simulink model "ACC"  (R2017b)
settings: Solver=FixedStepDiscrete  StartTime=0.0  StopTime=10.0  FixedStep=0.01  RelTol=1e-3  EnableMultiTasking=on
undefined symbols (not defined in the file): ACC_CONST0_NUMB, ACC_CONST1000_NUMB, ACC_CONST100_NUMB, ACC_CONST121_NUMB, ACC_CONST1_NUMB, ACC_CONST2047_NUMB, ACC_CONST60000_NUMB, ACC_CONST60_NUMB, ACC_CONSTF1_NUMB, ACC_RUNTIME_MS, ASWTYPE_FALSE, ASWTYPE_TRUE, CcACC_ACChrgDispSOCPrmt_pct, CcACC_ACChrgMismatch_ms, CcACC_ACChrgPACKVolLim_V, CcACC_ACChrgPACKVolLimTi_ms, CcACC_ACChrgPrmtObcFltLvl_numb, CcACC_ACChrgPrmtVcuFltLvl_numb, CcACC_ACChrgStepCurr_A, CcACC_ACChrgTempPrmtDelayTime_ms, CcACC_ACCrntUnctrolTi_ms, CcACC_ACFullChrgHysVolt_mV, CcACC_ACFullStepChrgTi1_ms, CcACC_ACFullStepChrgTi2_ms, CcACC_ACMaxChrgCurr_A, CcACC_ACStepChrgWaitTime_ms, CcACC_ACStop2DefaultTi_ms, CcACC_ACStop2DefaultTiDelay_ms, CcACC_BatFullResetTime_ms, CcACC_ChrgCrnt0HysVolt_mV, CcACC_ChrgEndDeviationVol1_mV, CcACC_ChrgEndDeviationVol2_mV, CcACC_ChrgEndDeviationVol3_mV, CcACC_ChrgMaxPackVoltLimt_V, CcACC_ChrgPwr1_W, CcACC_ChrgPwr2_W, CcACC_ChrgPwr3_W, CcACC_ChrgSt2StepChrgDeviVol_mV, CcACC_ChrgSt2StepChrgTime_ms, CcACC_ChrgStCutoffTime_ms, CcACC_ChrgStFullChrgCrnt_A, CcACC_CPDutyLowThrhd_pct, CcACC_CrntFilterTi1_cnt, CcACC_CrntFilterTi2_cnt, CcACC_CrntFilterTi2_ms, CcACC_CurrObcPreHeatLowThrhd_A, CcACC_DiffACChrgCrnt_A, CcACC_DiffACChrgCrntTi_ms, CcACC_DispSOCCalStart_pct, CcACC_DispSOCDiff_pct, CcACC_ElecLckRemTimeHold_ms, CcACC_HeatChrgCrnt0Time_ms, CcACC_HeatChrgCrnt1Time_ms, CcACC_Initial500Ti_ms, CcACC_Initial700Ti_ms, CcACC_MaxACChrgCellTemp_C, CcACC_MaxPackVoltLimt_V, CcACC_MinACChrgCellTemp_C, CcACC_MinACChrgCrntRqst_A, CcACC_OBCChrgPwr_W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
libraries: AIWAYS_Powertrain_BMS_lib x94, simulink x2
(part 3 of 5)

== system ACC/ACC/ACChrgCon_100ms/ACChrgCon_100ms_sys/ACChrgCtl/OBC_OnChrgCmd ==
  LbACC_ObcChrgCmd_flg : Inport
  GbADP_ChrgStopActive_flg : Inport  Port=2
  GeACC_ACChrgState_enum : Inport  Port=3
  GeUDS_AreaSel_enum : Inport  Port=4
  ACC_GbACC_ObcChrgCmd_flg : AIWAYS_Powertrain_BMS_lib/Signals/OverWrite  OverWrite_Value=CbACC_ObcChrgCmdOvr_flg  OverWrite_flag=CbACC_ObcChrgCmdOvrSwt_flg
  BMSDelay : AIWAYS_Powertrain_BMS_lib/Debounce & Delay/BMSDelay
  Constant1 : Constant  Value=ASWTYPE_FALSE
  Constant2 : Constant  Value=CcACC_ObcOnChrgCmdTi_ms
  Constant3 : Constant  Value=ASWTYPE_FALSE
  Constant4 : Constant  Value=Enum_ACCACChrgState.Enum_ACCACChrgState_Default
  Constant5 : Constant  Value=ACC_RUNTIME_MS
  Constant6 : Constant  Value=Enum_ACCACChrgState.Enum_ACCACChrgState_Stop
  Constant7 : Constant  Value=Enum_UDSAreaSel.Enum_UDSAreaSel_EU
  Constant8 : Constant  Value=ASWTYPE_FALSE
  Data Type Conversion1 : DataTypeConversion
  EdgeRising : AIWAYS_Powertrain_BMS_lib/Logical Operators/EdgeRising
  Logical Operator : Logic  Operator=OR  AllPortsSameDT=off  OutDataTypeStr=boolean
  Logical Operator1 : Logic  Operator=OR  Inputs=3  AllPortsSameDT=off  OutDataTypeStr=boolean
  Relational Operator1 : RelationalOperator  Operator===  OutDataTypeStr=boolean
  Relational Operator2 : RelationalOperator  Operator===  OutDataTypeStr=boolean
  Relational Operator3 : RelationalOperator  Operator===  OutDataTypeStr=boolean
  Switch : Switch  Criteria=u2 ~= 0  Threshold=1  RndMeth=Zero
  Switch1 : Switch  Criteria=u2 ~= 0  Threshold=1  RndMeth=Zero
  Switch3 : Switch  Criteria=u2 ~= 0  Threshold=1  RndMeth=Zero
  Unit Delay1 : UnitDelay  SampleTime=-1  StateName=StateName
  GbACC_ObcChrgCmd_flg : Outport
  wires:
  Unit Delay1/1 -> Switch3/3, BMSDelay/1
  Constant5/1 -> BMSDelay/2
  Constant2/1 -> BMSDelay/3
  LbACC_ObcChrgCmd_flg/1 -> Switch/3
  GbADP_ChrgStopActive_flg/1 -> Switch1/1
  EdgeRising/1 -> Logical Operator/1
  Constant1/1 -> Switch3/1
  Logical Operator/1 -> Switch/2, Unit Delay1/1
  Switch3/1 -> Logical Operator/2
  Constant3/1 -> Switch/1
  Constant4/1 -> Relational Operator1/2
  Constant6/1 -> Relational Operator2/2
  GeACC_ACChrgState_enum/1 -> Relational Operator1/1, Relational Operator2/1
  Relational Operator1/1 -> Logical Operator1/1
  Relational Operator2/1 -> Logical Operator1/2
  BMSDelay/1 -> Logical Operator1/3
  Logical Operator1/1 -> Switch3/2
  ACC_GbACC_ObcChrgCmd_flg/1 -> GbACC_ObcChrgCmd_flg/1  "GbACC_ObcChrgCmd_flg"
  Switch/1 -> ACC_GbACC_ObcChrgCmd_flg/1
  GeUDS_AreaSel_enum/1 -> Data Type Conversion1/1
  Data Type Conversion1/1 -> Relational Operator3/1
  Constant7/1 -> Relational Operator3/2
  Relational Operator3/1 -> Switch1/2
  Constant8/1 -> Switch1/3
  Switch1/1 -> EdgeRising/1

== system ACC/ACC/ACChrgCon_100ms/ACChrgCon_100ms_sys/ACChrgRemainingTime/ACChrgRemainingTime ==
  LcACC_FilterCrnt1_A : Inport
  GcHDP_PackCrnt_A : Inport  Port=2
  GcHDP_PackVolt_V : Inport  Port=3
  GeODP_ObcCcSt_enum : Inport  Port=4
  GcODP_ObcCpDuty_numb : Inport  Port=5
  GcVDP_ChrgLdReq_numb : Inport  Port=6
  GcODP_MaxPwrObcChrg_W : Inport  Port=7
  GeODP_ObcElecLck_enum : Inport  Port=8
  GcUDS_BatEnergy_kWh : Inport  Port=9
  GeUDS_CapSel_enum : Inport  Port=10
  GcSOC_DispSOC_pct : Inport  Port=11
  GcCDP_MaxCellVolt_mV : Inport  Port=12
  GcUDS_FullChrgCutoffVolt_mV : Inport  Port=13
  Enable : EnablePort  StatesWhenEnabling=reset
  ACChrgDeviationVolCorrect : Subsystem
  ACChrgRemainingTimePro : Subsystem
  BMSDebounceStartZero : AIWAYS_Powertrain_BMS_lib/Debounce & Delay/BMSDebounceStartZero
  ChrgRemainingTimeCalc : Subsystem
  Constant10 : Constant  Value=ACC_RUNTIME_MS
  Constant13 : Constant  Value=ACC_RUNTIME_MS
  Constant2 : Constant  Value=CcACC_ChrgStCutoffTime_ms
  Constant7 : Constant  Value=CcACC_ChrgStCutoffTime_ms
  Constant9 : Constant  Value=ACC_CONST100_NUMB
  Data Store Read2 : AIWAYS_Powertrain_BMS_lib/Signals/Data Store Read  Priority=0  DSR=EcNVM_ChrgPermitMaxSOC_pct
  Logical Operator : Logic  AllPortsSameDT=off  OutDataTypeStr=boolean
  Relational Operator1 : RelationalOperator  OutDataTypeStr=boolean
  Relational Operator3 : RelationalOperator  Operator===  OutDataTypeStr=boolean
  StepChrgRemainingTimeCalc : Subsystem
  Sum1 : Sum  Inputs=+-  OutDataTypeStr=Inherit: Inherit via back propagation  RndMeth=Zero
  Switch4 : Switch  Criteria=u2 ~= 0
  LcACC_ChrgingTiRem_min : Outport
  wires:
  ACChrgRemainingTimePro/1(LcACC_ChrgingTiRem_min) -> LcACC_ChrgingTiRem_min/1
  GcHDP_PackCrnt_A/1 -> ChrgRemainingTimeCalc/1(GcHDP_PackCrnt_A)
  LcACC_FilterCrnt1_A/1 -> ChrgRemainingTimeCalc/2(LcACC_FilterCrnt1_A)
  ChrgRemainingTimeCalc/1(LcACC_ChrgingTiRemCalc_min) -> Switch4/3
  GcHDP_PackVolt_V/1 -> ChrgRemainingTimeCalc/3(GcHDP_PackVolt_V)
  Logical Operator/1 -> StepChrgRemainingTimeCalc/Enable, Switch4/2
  StepChrgRemainingTimeCalc/1(LcACC_StepChrgTiRemCalc_min) -> Switch4/1
  Switch4/1 -> ACChrgRemainingTimePro/1(LcACC_TiRemCalc_min)
  GeODP_ObcCcSt_enum/1 -> ChrgRemainingTimeCalc/4(GeODP_ObcCcSt_enum)
  GcODP_ObcCpDuty_numb/1 -> ChrgRemainingTimeCalc/5(GcODP_ObcCpDuty_numb)
  GeODP_ObcElecLck_enum/1 -> ACChrgRemainingTimePro/2(GeODP_ObcElecLck_enum), ChrgRemainingTimeCalc/11(GeODP_ObcElecLck_enum)
  GcVDP_ChrgLdReq_numb/1 -> ChrgRemainingTimeCalc/6(GcVDP_ChrgLdReq_numb)
  GcUDS_BatEnergy_kWh/1 -> ChrgRemainingTimeCalc/8(GcUDS_BatEnergy_kWh)
  GeUDS_CapSel_enum/1 -> ChrgRemainingTimeCalc/9(GeUDS_CapSel_enum)
  GcSOC_DispSOC_pct/1 -> ChrgRemainingTimeCalc/10(GcSOC_DispSOC_pct)
  Constant9/1 -> Relational Operator3/2
  Data Store Read2/1 -> Relational Operator3/1
  Relational Operator3/1 -> Logical Operator/2
  GcCDP_MaxCellVolt_mV/1 -> Relational Operator1/1
  Sum1/1 -> Relational Operator1/2
  Constant2/1 -> BMSDebounceStartZero/2
  Constant13/1 -> BMSDebounceStartZero/5
  Constant10/1 -> BMSDebounceStartZero/3
  Relational Operator1/1 -> BMSDebounceStartZero/1
  Constant7/1 -> BMSDebounceStartZero/4
  BMSDebounceStartZero/1 -> Logical Operator/1
  GcODP_MaxPwrObcChrg_W/1 -> ACChrgDeviationVolCorrect/1(GcODP_MaxPwrObcChrg_W), ChrgRemainingTimeCalc/7(GcODP_MaxPwrObcChrg_W)
  GcUDS_FullChrgCutoffVolt_mV/1 -> Sum1/1
  ACChrgDeviationVolCorrect/1(LcACC_ChrgEndDeviationVol_mV) -> Sum1/2

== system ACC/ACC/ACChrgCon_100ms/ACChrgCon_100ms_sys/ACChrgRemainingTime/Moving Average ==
  note: Moving Average
  u : Inport
  R : Inport  Port=2  OutDataTypeStr=boolean
  Chart : Stateflow chart  TreatAsAtomicUnit=on
  Signal Conversion : SignalConversion  ConversionOutput=Contiguous copy  OverrideOpt=off
  y : Outport
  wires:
  Signal Conversion/1 -> y/1
  Chart/1(Y) -> Signal Conversion/1
  u/1 -> Chart/1(u)
  R/1 -> Chart/2(R)

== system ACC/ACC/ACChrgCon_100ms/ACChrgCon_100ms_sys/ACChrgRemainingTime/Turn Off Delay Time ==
  note: Turn Off Delay Time
  T : Inport
  u : Inport  Port=2
  dT : Inport  Port=3
  AND : Logic  Operator=OR  OutDataTypeStr=boolean
  Constant Value1 : Constant  Value=0  OutDataTypeStr=Inherit: Inherit via back propagation
  Constant Value2 : Constant  Value=0  OutDataTypeStr=Inherit: Inherit via back propagation
  EdgeFalling1 : Subsystem  Tag=R11-1  TreatAsAtomicUnit=on  mask(EdgeFalling){}
      mask help: The output indicates true if the logical input value changes from true to false. Input1=Value (u).
  Greater Than : RelationalOperator  Operator=>  OutDataTypeStr=boolean
  Minimum : MinMax  Function=max  Inputs=2
  Summation : Sum  Inputs=-+
  Switch : Switch  Criteria=u2 ~= 0  Threshold=1  RndMeth=Zero
  Unit Delay : UnitDelay  SampleTime=-1
  y : Outport
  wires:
  T/1 -> Switch/1
  EdgeFalling1/1(y) -> Switch/2
  Constant Value1/1 -> Minimum/2
  Summation/1 -> Minimum/1
  Constant Value2/1 -> Greater Than/2
  Unit Delay/1 -> Summation/2
  u/1 -> EdgeFalling1/1(u), AND/1
  AND/1 -> y/1
  Greater Than/1 -> AND/2
  Switch/1 -> Greater Than/1, Unit Delay/1
  dT/1 -> Summation/1
  Minimum/1 -> Switch/3

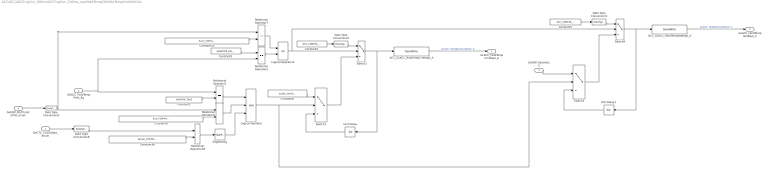
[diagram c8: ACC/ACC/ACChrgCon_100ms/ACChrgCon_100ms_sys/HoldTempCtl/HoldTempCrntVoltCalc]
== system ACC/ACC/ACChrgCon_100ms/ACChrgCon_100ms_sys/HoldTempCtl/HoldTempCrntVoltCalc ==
  GeCTC_CtrCtlState_enum : Inport
  GbACC_HoldTempPrmt_flg : Inport  Port=2
  GcHDP_PackVolt_V : Inport  Port=3
  GeVDP_PreThmVcuPmt_enum : Inport  Port=4
  ACC_GcACC_HoldTempCrntRqst_A : AIWAYS_Powertrain_BMS_lib/Signals/OverWrite  OverWrite_Value=CcACC_HoldTempCrntRqstOvr_A  OverWrite_flag=CbACC_HoldTempCrntRqstOvrSwt_flg
  ACC_GcACC_HoldTempVoltRqst_V : AIWAYS_Powertrain_BMS_lib/Signals/OverWrite  OverWrite_Value=CcACC_HoldTempVoltRqstOvr_V  OverWrite_flag=CbACC_HoldTempVoltRqstOvrSwt_flg
  Constant1 : Constant  Value=ASWTYPE_TRUE
  Constant10 : Constant  Value=Enum_VDPPreThmPmt.Enum_VDPPreThmPmt_HoldtempPmt
  Constant2 : Constant  Value=ACC_CONST0_NUMB
  Constant3 : Constant  Value=ASWTYPE_FALSE
  Constant36 : Constant  Value=Enum_CTCCtrCtlState.Enum_CTCCtrCtlState_Offline
  Constant5 : Constant  Value=ACC_CONST0_NUMB
  Constant8 : Constant  Value=CcACC_PreThmCrntRqst_A
  Constant9 : Constant  Value=Enum_VDPPreThmPmt.Enum_VDPPreThmPmt_HoldtempPmt
  Data Type Conversion{1..3,8} (4 alike) : DataTypeConversion
  EdgeRising : AIWAYS_Powertrain_BMS_lib/Logical Operators/EdgeRising
  Logical Operator : Logic  Inputs=3  AllPortsSameDT=off  OutDataTypeStr=boolean
  Logical Operator2 : Logic  Operator=OR  AllPortsSameDT=off  OutDataTypeStr=boolean
  Relational Operator{1..2,6,18} (4 alike) : RelationalOperator  Operator===  OutDataTypeStr=boolean
  Relational Operator7 : RelationalOperator  Operator=~=  OutDataTypeStr=boolean
  Switch{1..4} (4 alike) : Switch  Criteria=u2 ~= 0
  Unit Delay : UnitDelay  SampleTime=-1  StateName=StateName
  Unit Delay1 : UnitDelay  SampleTime=-1  StateName=StateName
  GcACC_HoldTempCrntRqst_A : Outport
  GcACC_HoldTempVoltRqst_V : Outport  Port=2
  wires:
  Relational Operator7/1 -> Logical Operator2/1
  Constant10/1 -> Relational Operator7/2
  Relational Operator6/1 -> Logical Operator/2
  Data Type Conversion3/1 -> Relational Operator7/1, Relational Operator6/1
  GeVDP_PreThmVcuPmt_enum/1 -> Data Type Conversion3/1
  Constant9/1 -> Relational Operator6/2
  Data Type Conversion1/1 -> Switch4/1
  Data Type Conversion2/1 -> Switch2/1
  Logical Operator2/1 -> Switch2/2, Switch4/2
  Relational Operator2/1 -> Logical Operator2/2
  GbACC_HoldTempPrmt_flg/1 -> Relational Operator2/2, Relational Operator1/1
  Constant3/1 -> Relational Operator2/1
  Data Type Conversion8/1 -> Relational Operator18/1
  Logical Operator/1 -> Switch1/2, Switch3/2
  Switch4/1 -> ACC_GcACC_HoldTempVoltRqst_V/1, Unit Delay1/1
  GcHDP_PackVolt_V/1 -> Switch3/1
  Switch3/1 -> Switch4/3
  Constant5/1 -> Data Type Conversion1/1
  Unit Delay1/1 -> Switch3/3
  GeCTC_CtrCtlState_enum/1 -> Data Type Conversion8/1
  Unit Delay/1 -> Switch1/3
  EdgeRising/1 -> Logical Operator/3
  Constant2/1 -> Data Type Conversion2/1
  Switch1/1 -> Switch2/3
  Constant8/1 -> Switch1/1
  Switch2/1 -> ACC_GcACC_HoldTempCrntRqst_A/1, Unit Delay/1
  Constant36/1 -> Relational Operator18/2
  Relational Operator1/1 -> Logical Operator/1
  Relational Operator18/1 -> EdgeRising/1
  Constant1/1 -> Relational Operator1/2
  ACC_GcACC_HoldTempCrntRqst_A/1 -> GcACC_HoldTempCrntRqst_A/1  "GcACC_HoldTempCrntRqst_A"
  ACC_GcACC_HoldTempVoltRqst_V/1 -> GcACC_HoldTempVoltRqst_V/1  "GcACC_HoldTempVoltRqst_V"

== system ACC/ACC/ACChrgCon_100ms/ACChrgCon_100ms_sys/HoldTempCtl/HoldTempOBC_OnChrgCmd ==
  GeVDP_PreThmVcuPmt_enum : Inport
  GbACC_HoldTempPrmt_flg : Inport  Port=2
  GeCTC_CtrCtlState_enum : Inport  Port=3
  ACC_GbACC_HoldTempObcChrgCmd_flg : AIWAYS_Powertrain_BMS_lib/Signals/OverWrite  OverWrite_Value=CbACC_HoldTempObcChrgCmdOvr_flg  OverWrite_flag=CbACC_HoldTempObcChrgCmdOvrSwt_flg
  BMSDelay : AIWAYS_Powertrain_BMS_lib/Debounce & Delay/BMSDelay
  Constant1 : Constant  Value=ASWTYPE_TRUE
  Constant18 : Constant  Value=CcACC_ObcCmdto1Ti_ms
  Constant2 : Constant  Value=ASWTYPE_FALSE
  Constant20 : Constant  Value=ACC_RUNTIME_MS
  Constant3 : Constant  Value=Enum_VDPPreThmPmt.Enum_VDPPreThmPmt_HoldtempPmt
  Constant36 : Constant  Value=Enum_CTCCtrCtlState.Enum_CTCCtrCtlState_Offline
  Constant4 : Constant  Value=ASWTYPE_FALSE
  Constant5 : Constant  Value=Enum_VDPPreThmPmt.Enum_VDPPreThmPmt_HoldtempPmt
  Constant8 : Constant  Value=ASWTYPE_TRUE
  Data Type Conversion2 : DataTypeConversion
  Data Type Conversion8 : DataTypeConversion
  EdgeRising : AIWAYS_Powertrain_BMS_lib/Logical Operators/EdgeRising
  Logical Operator : Logic  Inputs=3  AllPortsSameDT=off  OutDataTypeStr=boolean
  Logical Operator1 : Logic  Operator=OR  AllPortsSameDT=off  OutDataTypeStr=boolean
  Relational Operator{1,3..4,18} (4 alike) : RelationalOperator  Operator===  OutDataTypeStr=boolean
  Relational Operator2 : RelationalOperator  Operator=~=  OutDataTypeStr=boolean
  Switch1 : Switch  Criteria=u2 ~= 0
  Switch2 : Switch  Criteria=u2 ~= 0
  Unit Delay : UnitDelay  SampleTime=-1  StateName=StateName
  GbACC_HoldTempObcChrgCmd_flg : Outport
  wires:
  Relational Operator2/1 -> Logical Operator1/1
  Constant3/1 -> Relational Operator2/2
  Logical Operator1/1 -> Switch2/2
  Data Type Conversion2/1 -> Relational Operator4/1, Relational Operator2/1
  Constant5/1 -> Relational Operator4/2
  Relational Operator4/1 -> Logical Operator/2
  GeVDP_PreThmVcuPmt_enum/1 -> Data Type Conversion2/1
  BMSDelay/1 -> ACC_GbACC_HoldTempObcChrgCmd_flg/1
  Constant20/1 -> BMSDelay/2
  Constant18/1 -> BMSDelay/3
  Logical Operator/1 -> Switch1/2
  Constant4/1 -> Relational Operator3/1
  Unit Delay/1 -> Switch1/3
  Constant8/1 -> Switch1/1
  Constant2/1 -> Switch2/1
  Switch2/1 -> Unit Delay/1, BMSDelay/1
  Relational Operator3/1 -> Logical Operator1/2
  Switch1/1 -> Switch2/3
  EdgeRising/1 -> Logical Operator/3
  Relational Operator1/1 -> Logical Operator/1
  Relational Operator18/1 -> EdgeRising/1
  Data Type Conversion8/1 -> Relational Operator18/1
  GeCTC_CtrCtlState_enum/1 -> Data Type Conversion8/1
  Constant36/1 -> Relational Operator18/2
  GbACC_HoldTempPrmt_flg/1 -> Relational Operator3/2, Relational Operator1/1
  Constant1/1 -> Relational Operator1/2
  ACC_GbACC_HoldTempObcChrgCmd_flg/1 -> GbACC_HoldTempObcChrgCmd_flg/1  "GbACC_HoldTempObcChrgCmd_flg"

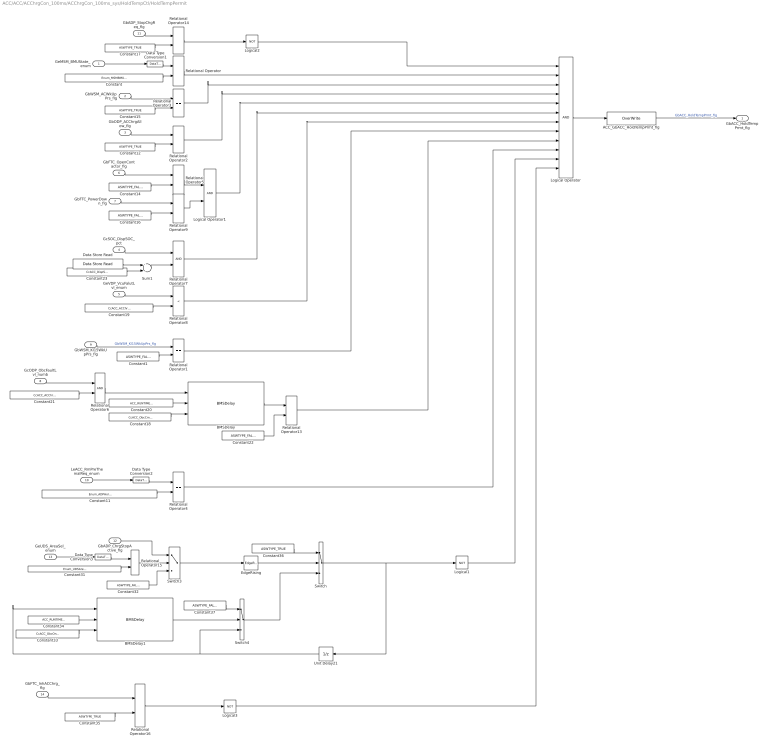
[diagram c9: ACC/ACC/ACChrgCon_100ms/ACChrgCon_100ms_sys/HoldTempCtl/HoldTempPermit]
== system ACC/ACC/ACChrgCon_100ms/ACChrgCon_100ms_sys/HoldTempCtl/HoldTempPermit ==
  GeMSM_BMUState_enum : Inport
  GbWSM_ACWkUpPrs_flg : Inport  Port=2
  GbODP_ACChrgAllow_flg : Inport  Port=3
  GcSOC_DispSOC_pct : Inport  Port=4
  GeVDP_VcuFalutLvl_enum : Inport  Port=5
  GbFTC_OpenContactor_flg : Inport  Port=6
  GbFTC_PowerDown_flg : Inport  Port=7
  GcODP_ObcFaultLvl_numb : Inport  Port=8
  GbWSM_Kl15WkUpPrs_flg : Inport  Port=9
  LeACC_RmPreThemalReq_enum : Inport  Port=10
  GbADP_StopChgReq_flg : Inport  Port=11
  GbADP_ChrgStopActive_flg : Inport  Port=12
  GeUDS_AreaSel_enum : Inport  Port=13
  GbFTC_InhACChrg_flg : Inport  Port=14
  ACC_GbACC_HoldTempPrmt_flg : AIWAYS_Powertrain_BMS_lib/Signals/OverWrite  OverWrite_Value=CbACC_HoldTempPrmtOvr_flg  OverWrite_flag=CbACC_HoldTempPrmtOvrSwt_flg
  BMSDelay : AIWAYS_Powertrain_BMS_lib/Debounce & Delay/BMSDelay
  BMSDelay1 : AIWAYS_Powertrain_BMS_lib/Debounce & Delay/BMSDelay
  Constant : Constant  Value=Enum_MSMBMUState.Enum_MSMBMUState_Run
  Constant{1,14,16,22,32,37} (6 alike) : Constant  Value=ASWTYPE_FALSE
  Constant11 : Constant  Value=Enum_ADPHoldtempReq.Enum_ADPHoldtempReq_HeatReq
  Constant{12,15,17,35..36} (5 alike) : Constant  Value=ASWTYPE_TRUE
  Constant18 : Constant  Value=CcACC_ObcCmdto0Ti_ms
  Constant19 : Constant  Value=CcACC_ACChrgPrmtVcuFltLvl_numb
  Constant20 : Constant  Value=ACC_RUNTIME_MS
  Constant21 : Constant  Value=CcACC_ACChrgPrmtObcFltLvl_numb
  Constant23 : Constant  Value=CcACC_DispSOCDiff_pct
  Constant31 : Constant  Value=Enum_UDSAreaSel.Enum_UDSAreaSel_EU
  Constant33 : Constant  Value=CcACC_ObcOnChrgCmdTi_ms
  Constant34 : Constant  Value=ACC_RUNTIME_MS
  Data Store Read : AIWAYS_Powertrain_BMS_lib/Signals/Data Store Read  Priority=0  DSR=EcNVM_ChrgPermitMaxSOC_pct
  Data Type Conversion1 : DataTypeConversion
  Data Type Conversion2 : DataTypeConversion
  Data Type Conversion3 : DataTypeConversion
  EdgeRising : AIWAYS_Powertrain_BMS_lib/Logical Operators/EdgeRising
  Logical Operator : Logic  Inputs=12  AllPortsSameDT=off  OutDataTypeStr=boolean
  Logical Operator1 : Logic  AllPortsSameDT=off  OutDataTypeStr=boolean
  Logical1 : Logic  Operator=NOT  OutDataTypeStr=boolean
  Logical2 : Logic  Operator=NOT  OutDataTypeStr=boolean
  Logical3 : Logic  Operator=NOT  OutDataTypeStr=boolean
  Relational Operator{,1..5,9,13..16} (11 alike) : RelationalOperator  Operator===  OutDataTypeStr=boolean
  Relational Operator6 : RelationalOperator  OutDataTypeStr=boolean
  Relational Operator7 : RelationalOperator  OutDataTypeStr=boolean
  Relational Operator8 : RelationalOperator  Operator=<  OutDataTypeStr=boolean
  Sum1 : Sum  Inputs=+-  OutDataTypeStr=Inherit: Inherit via back propagation  RndMeth=Zero
  Switch : Switch  Criteria=u2 ~= 0  Threshold=1  RndMeth=Zero
  Switch3 : Switch  Criteria=u2 ~= 0  Threshold=1  RndMeth=Zero
  Switch4 : Switch  Criteria=u2 ~= 0  Threshold=1  RndMeth=Zero
  Unit Delay21 : UnitDelay  SampleTime=-1  StateName=StateName
  GbACC_HoldTempPrmt_flg : Outport
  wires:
  Relational Operator13/1 -> Logical Operator/9
  GcODP_ObcFaultLvl_numb/1 -> Relational Operator6/1
  Constant21/1 -> Relational Operator6/2
  Constant18/1 -> BMSDelay/3
  BMSDelay/1 -> Relational Operator13/1
  Constant20/1 -> BMSDelay/2
  Constant22/1 -> Relational Operator13/2
  Relational Operator6/1 -> BMSDelay/1
  Constant16/1 -> Relational Operator9/2
  GbFTC_PowerDown_flg/1 -> Relational Operator9/1
  Relational Operator9/1 -> Logical Operator1/2
  Relational Operator5/1 -> Logical Operator1/1
  Logical Operator/1 -> ACC_GbACC_HoldTempPrmt_flg/1
  Relational Operator3/1 -> Logical Operator/3
  Constant/1 -> Relational Operator/2
  Relational Operator8/1 -> Logical Operator/7
  Constant14/1 -> Relational Operator5/2
  GbODP_ACChrgAllow_flg/1 -> Relational Operator2/1
  Data Type Conversion1/1 -> Relational Operator/1
  Relational Operator2/1 -> Logical Operator/4
  GeMSM_BMUState_enum/1 -> Data Type Conversion1/1
  Constant12/1 -> Relational Operator2/2
  Constant15/1 -> Relational Operator3/2
  GeVDP_VcuFalutLvl_enum/1 -> Relational Operator8/1
  GbFTC_OpenContactor_flg/1 -> Relational Operator5/1
  Sum1/1 -> Relational Operator7/2
  Logical Operator1/1 -> Logical Operator/5
  Relational Operator7/1 -> Logical Operator/6
  GcSOC_DispSOC_pct/1 -> Relational Operator7/1
  Constant19/1 -> Relational Operator8/2
  Relational Operator/1 -> Logical Operator/2
  GbWSM_ACWkUpPrs_flg/1 -> Relational Operator3/1
  GbWSM_Kl15WkUpPrs_flg/1 -> Relational Operator1/1  "GbWSM_Kl15WkUpPrs_flg"
  Constant1/1 -> Relational Operator1/2
  Relational Operator1/1 -> Logical Operator/8
  Constant11/1 -> Relational Operator4/2
  LeACC_RmPreThemalReq_enum/1 -> Data Type Conversion2/1
  Data Type Conversion2/1 -> Relational Operator4/1
  Relational Operator4/1 -> Logical Operator/10
  ACC_GbACC_HoldTempPrmt_flg/1 -> GbACC_HoldTempPrmt_flg/1  "GbACC_HoldTempPrmt_flg"
  Data Store Read/1 -> Sum1/1
  Constant23/1 -> Sum1/2
  Relational Operator14/1 -> Logical2/1
  GbADP_StopChgReq_flg/1 -> Relational Operator14/1
  Constant17/1 -> Relational Operator14/2
  Logical2/1 -> Logical Operator/1
  Logical1/1 -> Logical Operator/11
  Constant36/1 -> Switch/1
  Relational Operator15/1 -> Switch3/2
  EdgeRising/1 -> Switch/2
  Switch4/1 -> Switch/3
  Constant31/1 -> Relational Operator15/2
  GeUDS_AreaSel_enum/1 -> Data Type Conversion3/1
  Constant34/1 -> BMSDelay1/2
  Switch3/1 -> EdgeRising/1
  Constant32/1 -> Switch3/3
  Constant37/1 -> Switch4/1
  Data Type Conversion3/1 -> Relational Operator15/1
  Constant33/1 -> BMSDelay1/3
  Switch/1 -> Unit Delay21/1, Logical1/1
  Unit Delay21/1 -> Switch4/3, BMSDelay1/1
  BMSDelay1/1 -> Switch4/2
  GbADP_ChrgStopActive_flg/1 -> Switch3/1
  Constant35/1 -> Relational Operator16/2
  GbFTC_InhACChrg_flg/1 -> Relational Operator16/1
  Relational Operator16/1 -> Logical3/1
  Logical3/1 -> Logical Operator/12

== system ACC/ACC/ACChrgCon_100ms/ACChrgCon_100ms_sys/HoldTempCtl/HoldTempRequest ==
  GbACC_HoldTempPrmt_flg : Inport
  GeVDP_PreThmVcuPmt_enum : Inport  Port=2
  GeODP_ObcChrgSt_enum : Inport  Port=3
  ACC_GbACC_HoldTempRqst_flg : AIWAYS_Powertrain_BMS_lib/Signals/OverWrite  OverWrite_Value=CbACC_HoldTempRqstOvr_flg  OverWrite_flag=CbACC_HoldTempRqstOvrSwt_flg
  Constant1 : Constant  Value=Enum_ODPObcChrgSt.Enum_ODPObcChrgSt_WarmHeating
  Constant13 : Constant  Value=Enum_ODPObcChrgSt.Enum_ODPObcChrgSt_Ready
  Constant3 : Constant  Value=Enum_VDPPreThmPmt.Enum_VDPPreThmPmt_HoldtempPmt
  Constant5 : Constant  Value=ASWTYPE_TRUE
  Data Type Conversion2 : DataTypeConversion
  Data Type Conversion4 : DataTypeConversion
  Logical Operator : Logic  Inputs=3  AllPortsSameDT=off  OutDataTypeStr=boolean
  Logical Operator1 : Logic  Operator=OR  AllPortsSameDT=off  OutDataTypeStr=boolean
  Relational Operator{1..3,9} (4 alike) : RelationalOperator  Operator===  OutDataTypeStr=boolean
  GbACC_HoldTempRqst_flg : Outport
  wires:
  Logical Operator1/1 -> Logical Operator/3
  Relational Operator1/1 -> Logical Operator1/2
  Relational Operator9/1 -> Logical Operator1/1
  Constant1/1 -> Relational Operator1/2
  Logical Operator/1 -> ACC_GbACC_HoldTempRqst_flg/1
  Relational Operator2/1 -> Logical Operator/2
  Relational Operator3/1 -> Logical Operator/1
  Constant5/1 -> Relational Operator3/2
  Data Type Conversion4/1 -> Relational Operator1/1, Relational Operator9/1
  GeODP_ObcChrgSt_enum/1 -> Data Type Conversion4/1
  Constant13/1 -> Relational Operator9/2
  Data Type Conversion2/1 -> Relational Operator2/1
  GeVDP_PreThmVcuPmt_enum/1 -> Data Type Conversion2/1
  Constant3/1 -> Relational Operator2/2
  GbACC_HoldTempPrmt_flg/1 -> Relational Operator3/1
  ACC_GbACC_HoldTempRqst_flg/1 -> GbACC_HoldTempRqst_flg/1  "GbACC_HoldTempRqst_flg"

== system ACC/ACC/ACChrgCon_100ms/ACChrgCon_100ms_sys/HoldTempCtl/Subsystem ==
  GeADP_RmPreThemalReq_enum : Inport
  GcADP_RmPreThemalTime_min : Inport  Port=2
  BMSDelay : AIWAYS_Powertrain_BMS_lib/Debounce & Delay/BMSDelay
  Constant{1..2,6,10} (4 alike) : Constant  Value=Enum_ADPHoldtempReq.Enum_ADPHoldtempReq_HeatReq
  Constant3 : Constant  Value=Enum_ADPHoldtempReq.Enum_ADPHoldtempReq_Close
  Constant4 : Constant  Value=Enum_ADPHoldtempReq.Enum_ADPHoldtempReq_Close
  Constant5 : Constant  Value=ACC_RUNTIME_MS
  Constant7 : Constant  Value=ACC_CONST60000_NUMB
  Constant8 : Constant  Value=ASWTYPE_TRUE
  Data Type Conversion1 : DataTypeConversion
  Data Type Conversion2 : DataTypeConversion
  EdgeRising : AIWAYS_Powertrain_BMS_lib/Logical Operators/EdgeRising
  EdgeRising1 : AIWAYS_Powertrain_BMS_lib/Logical Operators/EdgeRising
  EdgeRising2 : AIWAYS_Powertrain_BMS_lib/Logical Operators/EdgeRising
  Logical Operator2 : Logic  Operator=OR  AllPortsSameDT=off  OutDataTypeStr=boolean
  Product5 : Product  OutDataTypeStr=Inherit: Inherit via back propagation
  Relational Operator{1..5} (5 alike) : RelationalOperator  Operator===  OutDataTypeStr=boolean
  Switch1 : Switch  Criteria=u2 ~= 0
  Switch2 : Switch  Criteria=u2 ~= 0
  Switch3 : Switch  Criteria=u2 ~= 0
  Unit Delay : UnitDelay  InitialCondition=Enum_ADPHoldtempReq.Enum_ADPHoldtempReq_NoRequest  SampleTime=-1  StateName=StateName
  Unit Delay1 : UnitDelay  InitialCondition=1  SampleTime=-1  StateName=StateName
  Unit Delay2 : UnitDelay  InitialCondition=Enum_ADPHoldtempReq.Enum_ADPHoldtempReq_NoRequest  SampleTime=-1  StateName=StateName
  LeACC_RmPreThemalReq_enum : Outport
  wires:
  Constant3/1 -> Relational Operator1/2
  EdgeRising/1 -> Switch3/2
  Constant1/1 -> Switch3/1
  Relational Operator4/1 -> EdgeRising/1
  EdgeRising1/1 -> Logical Operator2/1
  Constant4/1 -> Switch1/1
  Relational Operator1/1 -> EdgeRising1/1
  Constant2/1 -> Relational Operator4/2
  Data Type Conversion2/1 -> Relational Operator1/1, Relational Operator4/1
  GeADP_RmPreThemalReq_enum/1 -> Data Type Conversion2/1
  Switch1/1 -> Switch3/3
  Relational Operator2/1 -> BMSDelay/1
  Constant7/1 -> Product5/2
  Constant6/1 -> Relational Operator2/2
  EdgeRising2/1 -> Switch2/2
  Constant5/1 -> BMSDelay/2
  Unit Delay1/1 -> Switch2/3
  Switch2/1 -> Unit Delay1/1, Product5/1
  Product5/1 -> BMSDelay/3
  Relational Operator3/1 -> Logical Operator2/2
  Constant8/1 -> Relational Operator3/2
  BMSDelay/1 -> Relational Operator3/1
  Data Type Conversion1/1 -> LeACC_RmPreThemalReq_enum/1  "LeACC_RmPreThemalReq_enum"
  Switch3/1 -> Unit Delay2/1, Unit Delay/1, Data Type Conversion1/1
  GcADP_RmPreThemalTime_min/1 -> Switch2/1
  Constant10/1 -> Relational Operator5/2
  Relational Operator5/1 -> EdgeRising2/1
  Unit Delay2/1 -> Relational Operator2/1, Relational Operator5/1
  Logical Operator2/1 -> Switch1/2
  Unit Delay/1 -> Switch1/3

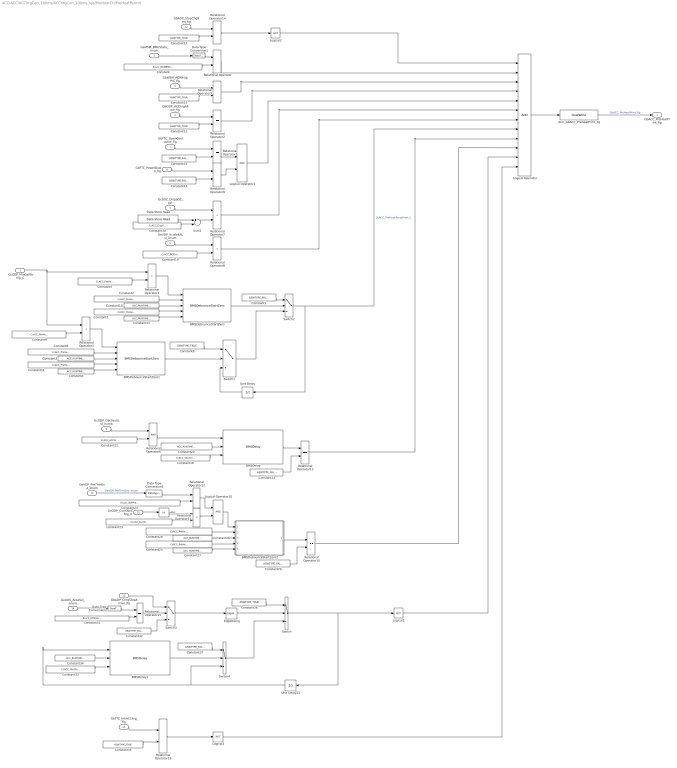
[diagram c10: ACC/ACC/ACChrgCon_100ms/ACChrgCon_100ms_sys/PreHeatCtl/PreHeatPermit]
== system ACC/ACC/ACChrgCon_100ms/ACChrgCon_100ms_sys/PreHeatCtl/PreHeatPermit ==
  GcCDP_MinCellTemp_C : Inport
  GeMSM_BMUState_enum : Inport  Port=2
  GbWSM_ACWkUpPrs_flg : Inport  Port=3
  GbODP_ACChrgAllow_flg : Inport  Port=4
  GcSOC_DispSOC_pct : Inport  Port=5
  GeVDP_VcuFalutLvl_enum : Inport  Port=6
  GbFTC_OpenContactor_flg : Inport  Port=7
  GbFTC_PowerDown_flg : Inport  Port=8
  GcODP_ObcFaultLvl_numb : Inport  Port=9
  GeVDP_PreThmEna_enum : Inport  Port=10
  GcODP_CurrObcChrg_A : Inport  Port=11
  GbADP_StopChgReq_flg : Inport  Port=12
  GbADP_ChrgStopActive_flg : Inport  Port=13
  GeUDS_AreaSel_enum : Inport  Port=14
  GbFTC_InhACChrg_flg : Inport  Port=15
  ACC_GbACC_PreHeatPrmt_flg : AIWAYS_Powertrain_BMS_lib/Signals/OverWrite  OverWrite_Value=CbACC_PreHeatPrmtOvr_flg  OverWrite_flag=CbACC_PreHeatPrmtOvrSwt_flg
  Abs : Abs
  BMSDebounceStartZero : AIWAYS_Powertrain_BMS_lib/Debounce & Delay/BMSDebounceStartZero
  BMSDebounceStartZero1 : AIWAYS_Powertrain_BMS_lib/Debounce & Delay/BMSDebounceStartZero
  BMSDebounceStartZero2 : Subsystem  TreatAsAtomicUnit=on  mask(Debounce){}
      mask help: Note: The maximum of Heal2Fault and Fault2Heal is 600000; Description: The counter of debounce start from zero. 1. When FaultFlag is false and signl is ture, the Heal2Fault counter increase until it reach to Heal2Fault value, then set FaultFlag to true; 2. When FaultFlag is false and signl is false, the Heal2Fault counter decrease until it reach to zero; 3. When FaultFlag is ture and signl is false, the Fault2Heal counter increase until it reach to Fault2Heal value, then set FaultFlag to false; 4. When FaultFlag is ture and signl is ture, the Fault2Heal counter decrease until it reach to zero;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
  BMSDelay : AIWAYS_Powertrain_BMS_lib/Debounce & Delay/BMSDelay
  BMSDelay1 : AIWAYS_Powertrain_BMS_lib/Debounce & Delay/BMSDelay
  Constant : Constant  Value=Enum_MSMBMUState.Enum_MSMBMUState_Run
  Constant{1,14,16,22,29,32,37} (7 alike) : Constant  Value=ASWTYPE_FALSE
  Constant{3..4,10,13,20,26..27,34} (8 alike) : Constant  Value=ACC_RUNTIME_MS
  Constant{2,6..7,11} (4 alike) : Constant  Value=CcACC_PreHeatTempPrmtDelayTime_ms
  Constant{8,12,15,17,35..36} (6 alike) : Constant  Value=ASWTYPE_TRUE
  Constant18 : Constant  Value=CcACC_ObcCmdto0Ti_ms
  Constant19 : Constant  Value=CcACC_ACChrgPrmtVcuFltLvl_numb
  Constant21 : Constant  Value=CcACC_ACChrgPrmtObcFltLvl_numb
  Constant23 : Constant  Value=CcACC_CurrObcPreHeatLowThrhd_A
  Constant24 : Constant  Value=Enum_VDPPreThmEna.Enum_VDPPreThmEna_PreHeatEna
  Constant25 : Constant  Value=CcACC_PreHeatPTCFailDelayTi_ms
  Constant28 : Constant  Value=CcACC_PreHeatPTCFailDelayTi_ms
  Constant30 : Constant  Value=CcACC_DispSOCDiff_pct
  Constant31 : Constant  Value=Enum_UDSAreaSel.Enum_UDSAreaSel_EU
  Constant33 : Constant  Value=CcACC_ObcOnChrgCmdTi_ms
  Constant5 : Constant  Value=CcACC_PreHeatUpLmt_C
  Constant9 : Constant  Value=CcACC_PreHeatDwnLmt_C
  Data Store Read : AIWAYS_Powertrain_BMS_lib/Signals/Data Store Read  Priority=0  DSR=EcNVM_ChrgPermitMaxSOC_pct
  Data Type Conversion1 : DataTypeConversion
  Data Type Conversion2 : DataTypeConversion
  Data Type Conversion5 : DataTypeConversion
  EdgeRising : AIWAYS_Powertrain_BMS_lib/Logical Operators/EdgeRising
  Logical Operator : Logic  Inputs=12  AllPortsSameDT=off  OutDataTypeStr=boolean
  Logical Operator1 : Logic  AllPortsSameDT=off  OutDataTypeStr=boolean
  Logical Operator10 : Logic  AllPortsSameDT=off  OutDataTypeStr=boolean
  Logical1 : Logic  Operator=NOT  OutDataTypeStr=boolean
  Logical2 : Logic  Operator=NOT  OutDataTypeStr=boolean
  Logical3 : Logic  Operator=NOT  OutDataTypeStr=boolean
  Relational Operator{,2..3,5,9..10,12..16} (11 alike) : RelationalOperator  Operator===  OutDataTypeStr=boolean
  Relational Operator{1,7..8,11} (4 alike) : RelationalOperator  Operator=<  OutDataTypeStr=boolean
  Relational Operator4 : RelationalOperator  Operator=>  OutDataTypeStr=boolean
  Relational Operator6 : RelationalOperator  OutDataTypeStr=boolean
  Sum1 : Sum  Inputs=+-  OutDataTypeStr=Inherit: Inherit via back propagation  RndMeth=Zero
  Switch : Switch  Criteria=u2 ~= 0  Threshold=1  RndMeth=Zero
  Switch1 : Switch  Criteria=u2 ~= 0
  Switch2 : Switch  Criteria=u2 ~= 0
  Switch3 : Switch  Criteria=u2 ~= 0  Threshold=1  RndMeth=Zero
  Switch4 : Switch  Criteria=u2 ~= 0  Threshold=1  RndMeth=Zero
  Unit Delay : UnitDelay  SampleTime=-1  StateName=StateName
  Unit Delay21 : UnitDelay  SampleTime=-1  StateName=StateName
  GbACC_PreHeatPrmt_flg : Outport
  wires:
  Constant9/1 -> Relational Operator1/2
  Constant11/1 -> BMSDebounceStartZero1/4
  Constant3/1 -> BMSDebounceStartZero1/3
  Constant4/1 -> BMSDebounceStartZero1/5
  Constant6/1 -> BMSDebounceStartZero1/2
  Relational Operator1/1 -> BMSDebounceStartZero1/1
  Relational Operator4/1 -> BMSDebounceStartZero/1
  Constant2/1 -> BMSDebounceStartZero/2
  Constant13/1 -> BMSDebounceStartZero/5
  Constant10/1 -> BMSDebounceStartZero/3
  Constant7/1 -> BMSDebounceStartZero/4
  GcCDP_MinCellTemp_C/1 -> Relational Operator4/1, Relational Operator1/1
  Constant5/1 -> Relational Operator4/2
  Unit Delay/1 -> Switch1/3
  Constant8/1 -> Switch1/1
  BMSDebounceStartZero1/1 -> Switch1/2
  Switch1/1 -> Switch2/3
  Constant1/1 -> Switch2/1
  BMSDebounceStartZero/1 -> Switch2/2
  GbWSM_ACWkUpPrs_flg/1 -> Relational Operator3/1
  Relational Operator/1 -> Logical Operator/2
  Constant19/1 -> Relational Operator8/2
  GcSOC_DispSOC_pct/1 -> Relational Operator7/1
  Relational Operator7/1 -> Logical Operator/6
  Logical Operator1/1 -> Logical Operator/5
  Sum1/1 -> Relational Operator7/2
  GbFTC_OpenContactor_flg/1 -> Relational Operator5/1
  GeVDP_VcuFalutLvl_enum/1 -> Relational Operator8/1
  Constant15/1 -> Relational Operator3/2
  Constant12/1 -> Relational Operator2/2
  GeMSM_BMUState_enum/1 -> Data Type Conversion1/1
  Relational Operator2/1 -> Logical Operator/4
  Data Type Conversion1/1 -> Relational Operator/1
  Switch2/1 -> Logical Operator/8, Unit Delay/1  "LbACC_PreHeatTempPrmt_flg"
  GbODP_ACChrgAllow_flg/1 -> Relational Operator2/1
  Constant14/1 -> Relational Operator5/2
  Relational Operator8/1 -> Logical Operator/7
  Constant/1 -> Relational Operator/2
  Relational Operator3/1 -> Logical Operator/3
  Logical Operator/1 -> ACC_GbACC_PreHeatPrmt_flg/1
  ACC_GbACC_PreHeatPrmt_flg/1 -> GbACC_PreHeatPrmt_flg/1  "GbACC_PreHeatPrmt_flg"
  Relational Operator5/1 -> Logical Operator1/1
  Relational Operator9/1 -> Logical Operator1/2
  GbFTC_PowerDown_flg/1 -> Relational Operator9/1
  Constant16/1 -> Relational Operator9/2
  Relational Operator6/1 -> BMSDelay/1
  Constant22/1 -> Relational Operator13/2
  Constant20/1 -> BMSDelay/2
  BMSDelay/1 -> Relational Operator13/1
  Constant18/1 -> BMSDelay/3
  Constant21/1 -> Relational Operator6/2
  GcODP_ObcFaultLvl_numb/1 -> Relational Operator6/1
  Relational Operator13/1 -> Logical Operator/9
  Relational Operator12/1 -> Logical Operator10/1
  Constant27/1 -> BMSDebounceStartZero2/5(HealStep)
  Constant28/1 -> BMSDebounceStartZero2/2(Hearl2Fault)
  Relational Operator11/1 -> Logical Operator10/2
  Data Type Conversion5/1 -> Relational Operator12/1
  Abs/1 -> Relational Operator11/1
  GcODP_CurrObcChrg_A/1 -> Abs/1
  GeVDP_PreThmEna_enum/1 -> Data Type Conversion5/1  "GeVDP_PreThmEna_enum"
  Constant26/1 -> BMSDebounceStartZero2/3(FaultStep)
  Constant25/1 -> BMSDebounceStartZero2/4(Fault2Heal)
  Logical Operator10/1 -> BMSDebounceStartZero2/1(Signal)
  Constant24/1 -> Relational Operator12/2
  Constant23/1 -> Relational Operator11/2
  Constant29/1 -> Relational Operator10/2
  BMSDebounceStartZero2/1(FaultFlag) -> Relational Operator10/1
  Relational Operator10/1 -> Logical Operator/10
  Data Store Read/1 -> Sum1/1
  Constant30/1 -> Sum1/2
  GbADP_StopChgReq_flg/1 -> Relational Operator14/1
  Constant17/1 -> Relational Operator14/2
  Relational Operator14/1 -> Logical2/1
  Logical2/1 -> Logical Operator/1
  Constant36/1 -> Switch/1
  Relational Operator15/1 -> Switch3/2
  EdgeRising/1 -> Switch/2
  Switch4/1 -> Switch/3
  Constant31/1 -> Relational Operator15/2
  GeUDS_AreaSel_enum/1 -> Data Type Conversion2/1
  Unit Delay21/1 -> Switch4/3, BMSDelay1/1
  Logical1/1 -> Logical Operator/11
  Constant34/1 -> BMSDelay1/2
  Switch3/1 -> EdgeRising/1
  Constant33/1 -> BMSDelay1/3
  Constant32/1 -> Switch3/3
  Data Type Conversion2/1 -> Relational Operator15/1
  Constant37/1 -> Switch4/1
  GbADP_ChrgStopActive_flg/1 -> Switch3/1
  Switch/1 -> Unit Delay21/1, Logical1/1
  BMSDelay1/1 -> Switch4/2
  Constant35/1 -> Relational Operator16/2
  GbFTC_InhACChrg_flg/1 -> Relational Operator16/1
  Relational Operator16/1 -> Logical3/1
  Logical3/1 -> Logical Operator/12

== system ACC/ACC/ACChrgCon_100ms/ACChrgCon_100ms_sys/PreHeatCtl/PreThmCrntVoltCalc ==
  GeCTC_CtrCtlState_enum : Inport
  GbACC_PreHeatPrmt_flg : Inport  Port=2
  GcHDP_PackVolt_V : Inport  Port=3
  GeVDP_PreThmVcuPmt_enum : Inport  Port=4
  ACC_GcACC_PreThmCrntRqst_A : AIWAYS_Powertrain_BMS_lib/Signals/OverWrite  OverWrite_Value=CcACC_PreThmCrntRqstOvr_A  OverWrite_flag=CbACC_PreThmCrntRqstOvrSwt_flg
  ACC_GcACC_PreThmVoltRqst_V : AIWAYS_Powertrain_BMS_lib/Signals/OverWrite  OverWrite_Value=CcACC_PreThmVoltRqstOvr_V  OverWrite_flag=CbACC_PreThmVoltRqstOvrSwt_flg
  Constant1 : Constant  Value=ASWTYPE_TRUE
  Constant10 : Constant  Value=Enum_VDPPreThmPmt.Enum_VDPPreThmPmt_PreHeatPmt
  Constant2 : Constant  Value=ACC_CONST0_NUMB
  Constant3 : Constant  Value=ASWTYPE_FALSE
  Constant36 : Constant  Value=Enum_CTCCtrCtlState.Enum_CTCCtrCtlState_Offline
  Constant5 : Constant  Value=ACC_CONST0_NUMB
  Constant8 : Constant  Value=CcACC_PreThmCrntRqst_A
  Constant9 : Constant  Value=Enum_VDPPreThmPmt.Enum_VDPPreThmPmt_PreHeatPmt
  Data Type Conversion{1..3,8} (4 alike) : DataTypeConversion
  EdgeRising : AIWAYS_Powertrain_BMS_lib/Logical Operators/EdgeRising
  Logical Operator : Logic  Inputs=3  AllPortsSameDT=off  OutDataTypeStr=boolean
  Logical Operator2 : Logic  Operator=OR  AllPortsSameDT=off  OutDataTypeStr=boolean
  Relational Operator{1..2,6,18} (4 alike) : RelationalOperator  Operator===  OutDataTypeStr=boolean
  Relational Operator7 : RelationalOperator  Operator=~=  OutDataTypeStr=boolean
  Switch{1..4} (4 alike) : Switch  Criteria=u2 ~= 0
  Unit Delay : UnitDelay  SampleTime=-1  StateName=StateName
  Unit Delay1 : UnitDelay  SampleTime=-1  StateName=StateName
  GcACC_PreThmCrntRqst_A : Outport
  GcACC_PreThmVoltRqst_V : Outport  Port=2
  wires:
  Constant1/1 -> Relational Operator1/2
  Relational Operator18/1 -> EdgeRising/1
  Relational Operator1/1 -> Logical Operator/1
  Constant36/1 -> Relational Operator18/2
  Switch2/1 -> ACC_GcACC_PreThmCrntRqst_A/1, Unit Delay/1
  Constant8/1 -> Switch1/1
  Switch1/1 -> Switch2/3
  Constant2/1 -> Data Type Conversion2/1
  EdgeRising/1 -> Logical Operator/3
  Unit Delay/1 -> Switch1/3
  GeCTC_CtrCtlState_enum/1 -> Data Type Conversion8/1
  Unit Delay1/1 -> Switch3/3
  Constant5/1 -> Data Type Conversion1/1
  Switch3/1 -> Switch4/3
  GcHDP_PackVolt_V/1 -> Switch3/1
  Switch4/1 -> Unit Delay1/1, ACC_GcACC_PreThmVoltRqst_V/1
  Logical Operator/1 -> Switch3/2, Switch1/2
  Data Type Conversion8/1 -> Relational Operator18/1
  Constant3/1 -> Relational Operator2/1
  GbACC_PreHeatPrmt_flg/1 -> Relational Operator1/1, Relational Operator2/2
  Relational Operator2/1 -> Logical Operator2/2
  Logical Operator2/1 -> Switch4/2, Switch2/2
  ACC_GcACC_PreThmCrntRqst_A/1 -> GcACC_PreThmCrntRqst_A/1  "GcACC_PreThmCrntRqst_A"
  ACC_GcACC_PreThmVoltRqst_V/1 -> GcACC_PreThmVoltRqst_V/1  "GcACC_PreThmVoltRqst_V"
  Data Type Conversion2/1 -> Switch2/1
  Data Type Conversion1/1 -> Switch4/1
  Constant9/1 -> Relational Operator6/2
  GeVDP_PreThmVcuPmt_enum/1 -> Data Type Conversion3/1
  Data Type Conversion3/1 -> Relational Operator6/1, Relational Operator7/1
  Relational Operator6/1 -> Logical Operator/2
  Constant10/1 -> Relational Operator7/2
  Relational Operator7/1 -> Logical Operator2/1

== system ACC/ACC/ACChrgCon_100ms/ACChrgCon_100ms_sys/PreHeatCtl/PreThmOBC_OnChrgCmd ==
  GeVDP_PreThmVcuPmt_enum : Inport
  GbACC_PreHeatPrmt_flg : Inport  Port=2
  GeCTC_CtrCtlState_enum : Inport  Port=3
  ACC_GbACC_PreThmObcChrgCmd_flg : AIWAYS_Powertrain_BMS_lib/Signals/OverWrite  OverWrite_Value=CbACC_PreThmObcChrgCmdOvr_flg  OverWrite_flag=CbACC_PreThmObcChrgCmdOvrSwt_flg
  BMSDelay : AIWAYS_Powertrain_BMS_lib/Debounce & Delay/BMSDelay
  Constant1 : Constant  Value=ASWTYPE_TRUE
  Constant18 : Constant  Value=CcACC_ObcCmdto1Ti_ms
  Constant2 : Constant  Value=ASWTYPE_FALSE
  Constant20 : Constant  Value=ACC_RUNTIME_MS
  Constant3 : Constant  Value=Enum_VDPPreThmPmt.Enum_VDPPreThmPmt_PreHeatPmt
  Constant36 : Constant  Value=Enum_CTCCtrCtlState.Enum_CTCCtrCtlState_Offline
  Constant4 : Constant  Value=ASWTYPE_FALSE
  Constant5 : Constant  Value=Enum_VDPPreThmPmt.Enum_VDPPreThmPmt_PreHeatPmt
  Constant8 : Constant  Value=ASWTYPE_TRUE
  Data Type Conversion2 : DataTypeConversion
  Data Type Conversion8 : DataTypeConversion
  EdgeRising : AIWAYS_Powertrain_BMS_lib/Logical Operators/EdgeRising
  Logical Operator : Logic  Inputs=3  AllPortsSameDT=off  OutDataTypeStr=boolean
  Logical Operator1 : Logic  Operator=OR  AllPortsSameDT=off  OutDataTypeStr=boolean
  Relational Operator{1,3..4,18} (4 alike) : RelationalOperator  Operator===  OutDataTypeStr=boolean
  Relational Operator2 : RelationalOperator  Operator=~=  OutDataTypeStr=boolean
  Switch1 : Switch  Criteria=u2 ~= 0
  Switch2 : Switch  Criteria=u2 ~= 0
  Unit Delay : UnitDelay  SampleTime=-1  StateName=StateName
  GbACC_PreThmObcChrgCmd_flg : Outport
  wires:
  Constant1/1 -> Relational Operator1/2
  GbACC_PreHeatPrmt_flg/1 -> Relational Operator1/1, Relational Operator3/2
  Constant36/1 -> Relational Operator18/2
  GeCTC_CtrCtlState_enum/1 -> Data Type Conversion8/1
  Data Type Conversion8/1 -> Relational Operator18/1
  Relational Operator18/1 -> EdgeRising/1
  Relational Operator1/1 -> Logical Operator/1
  EdgeRising/1 -> Logical Operator/3
  Switch1/1 -> Switch2/3
  Relational Operator3/1 -> Logical Operator1/2
  Switch2/1 -> BMSDelay/1, Unit Delay/1
  Constant2/1 -> Switch2/1
  Constant8/1 -> Switch1/1
  Unit Delay/1 -> Switch1/3
  Constant4/1 -> Relational Operator3/1
  ACC_GbACC_PreThmObcChrgCmd_flg/1 -> GbACC_PreThmObcChrgCmd_flg/1  "GbACC_PreThmObcChrgCmd_flg"
  Logical Operator/1 -> Switch1/2
  Constant18/1 -> BMSDelay/3
  Constant20/1 -> BMSDelay/2
  BMSDelay/1 -> ACC_GbACC_PreThmObcChrgCmd_flg/1
  GeVDP_PreThmVcuPmt_enum/1 -> Data Type Conversion2/1
  Relational Operator4/1 -> Logical Operator/2
  Constant5/1 -> Relational Operator4/2
  Data Type Conversion2/1 -> Relational Operator2/1, Relational Operator4/1
  Logical Operator1/1 -> Switch2/2
  Constant3/1 -> Relational Operator2/2
  Relational Operator2/1 -> Logical Operator1/1

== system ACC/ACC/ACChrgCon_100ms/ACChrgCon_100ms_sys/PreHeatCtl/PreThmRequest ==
  GbACC_PreHeatPrmt_flg : Inport
  GeVDP_PreThmVcuPmt_enum : Inport  Port=2
  GeODP_ObcChrgSt_enum : Inport  Port=3
  ACC_GbACC_PreThmRqst_flg : AIWAYS_Powertrain_BMS_lib/Signals/OverWrite  OverWrite_Value=CbACC_PreThmRqstOvr_flg  OverWrite_flag=CbACC_PreThmRqstOvrSwt_flg
  Constant1 : Constant  Value=Enum_ODPObcChrgSt.Enum_ODPObcChrgSt_PreHeating
  Constant13 : Constant  Value=Enum_ODPObcChrgSt.Enum_ODPObcChrgSt_Ready
  Constant3 : Constant  Value=Enum_VDPPreThmPmt.Enum_VDPPreThmPmt_PreHeatPmt
  Constant5 : Constant  Value=ASWTYPE_TRUE
  Data Type Conversion2 : DataTypeConversion
  Data Type Conversion4 : DataTypeConversion
  Logical Operator : Logic  Inputs=3  AllPortsSameDT=off  OutDataTypeStr=boolean
  Logical Operator1 : Logic  Operator=OR  AllPortsSameDT=off  OutDataTypeStr=boolean
  Relational Operator{1..3,9} (4 alike) : RelationalOperator  Operator===  OutDataTypeStr=boolean
  GbACC_PreThmRqst_flg : Outport
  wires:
  GbACC_PreHeatPrmt_flg/1 -> Relational Operator3/1
  Constant3/1 -> Relational Operator2/2
  GeVDP_PreThmVcuPmt_enum/1 -> Data Type Conversion2/1
  Data Type Conversion2/1 -> Relational Operator2/1
  Constant13/1 -> Relational Operator9/2
  GeODP_ObcChrgSt_enum/1 -> Data Type Conversion4/1
  Data Type Conversion4/1 -> Relational Operator9/1, Relational Operator1/1
  Constant5/1 -> Relational Operator3/2
  Relational Operator3/1 -> Logical Operator/1
  Relational Operator2/1 -> Logical Operator/2
  Logical Operator/1 -> ACC_GbACC_PreThmRqst_flg/1
  ACC_GbACC_PreThmRqst_flg/1 -> GbACC_PreThmRqst_flg/1  "GbACC_PreThmRqst_flg"
  Constant1/1 -> Relational Operator1/2
  Relational Operator9/1 -> Logical Operator1/1
  Relational Operator1/1 -> Logical Operator1/2
  Logical Operator1/1 -> Logical Operator/3

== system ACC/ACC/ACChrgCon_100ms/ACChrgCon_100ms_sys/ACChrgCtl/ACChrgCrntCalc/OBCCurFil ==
  OBC_MaxCur : Inport
  Last_CurReq : Inport  Port=2
  BMSDelay3 : AIWAYS_Powertrain_BMS_lib/Debounce & Delay/BMSDelay
  Constant1 : Constant  Value=ACC_CONST0_NUMB
  Constant12 : Constant  Value=CcACC_OBCCurFilterLim_A
  Constant14 : Constant  Value=ACC_RUNTIME_MS  OutDataTypeStr=uint8
  Constant20 : Constant  Value=CcACC_OBCCurFilterTi_ms  OutDataTypeStr=uint16
  Data Type Conversion : DataTypeConversion  OutDataTypeStr=single
  EdgeRising : AIWAYS_Powertrain_BMS_lib/Logical Operators/EdgeRising
  Logical : Logic  OutDataTypeStr=boolean
  Logical1 : Logic  Operator=NOT  OutDataTypeStr=boolean
  Logical2 : Logic  Operator=OR  OutDataTypeStr=boolean
  Logical4 : Logic  Operator=NOT  OutDataTypeStr=boolean
  Relational Operator1 : RelationalOperator  Operator=>  OutDataTypeStr=boolean
  Relational Operator7 : RelationalOperator  OutDataTypeStr=boolean
  Subsystem : Subsystem
  Sum3 : Sum  Inputs=+-  OutDataTypeStr=Inherit: Inherit via back propagation  RndMeth=Zero
  Switch8 : Switch  Criteria=u2 ~= 0  Threshold=1  RndMeth=Zero
  Switch9 : Switch  Criteria=u2 ~= 0  Threshold=1  RndMeth=Zero
  Unit Delay1 : UnitDelay  SampleTime=-1  StateName=StateName
  CurReqFil : Outport
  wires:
  Switch8/1 -> CurReqFil/1
  OBC_MaxCur/1 -> Switch9/1, Switch8/1, Sum3/1
  Constant14/1 -> BMSDelay3/2
  Switch9/1 -> Switch8/3
  Relational Operator7/1 -> Logical4/1, Switch8/2
  Constant12/1 -> Relational Operator7/2
  BMSDelay3/1 -> Unit Delay1/1, Switch9/2
  Sum3/1 -> Relational Operator1/1, Relational Operator7/1
  Logical4/1 -> Logical/1
  Last_CurReq/1 -> Sum3/2, Switch9/3
  Constant20/1 -> BMSDelay3/3
  Subsystem/1(Q) -> BMSDelay3/1
  EdgeRising/1 -> Logical2/2
  Logical/1 -> Logical1/1, Subsystem/1(set)
  Constant1/1 -> Data Type Conversion/1
  Unit Delay1/1 -> EdgeRising/1
  Relational Operator1/1 -> Logical/2
  Data Type Conversion/1 -> Relational Operator1/2
  Logical1/1 -> Logical2/1
  Logical2/1 -> Subsystem/2(clear)

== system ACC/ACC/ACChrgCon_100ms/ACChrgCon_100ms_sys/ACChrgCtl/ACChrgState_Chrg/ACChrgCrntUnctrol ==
  GcCDP_MaxCellVolt_mV : Inport
  GcUDS_FullChrgCutoffVolt_mV : Inport  Port=2
  ACC_GbACC_ACCrntUnctrolFlt_flg : AIWAYS_Powertrain_BMS_lib/Signals/OverWrite  OverWrite_Value=CbACC_ACCrntUnctrolFltOvr_flg  OverWrite_flag=CbACC_ACCrntUnctrolFltOvrSwt_flg
  Add : Sum
  BMSDebounceStartZero : AIWAYS_Powertrain_BMS_lib/Debounce & Delay/BMSDebounceStartZero
  Constant10 : Constant  Value=CcACC_ACFullChrgHysVolt_mV
  Constant13 : Constant  Value=ACC_RUNTIME_MS
  Constant2 : Constant  Value=CcACC_ACCrntUnctrolTi_ms
  Constant3 : Constant  Value=ACC_RUNTIME_MS
  Constant9 : Constant  Value=CcACC_ACCrntUnctrolTi_ms
  Relational Operator4 : RelationalOperator  OutDataTypeStr=boolean
  GbACC_ACCrntUnctrolFlt_flg : Outport
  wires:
  GcCDP_MaxCellVolt_mV/1 -> Relational Operator4/1
  Add/1 -> Relational Operator4/2
  Constant10/1 -> Add/2
  GcUDS_FullChrgCutoffVolt_mV/1 -> Add/1
  Relational Operator4/1 -> BMSDebounceStartZero/1
  ACC_GbACC_ACCrntUnctrolFlt_flg/1 -> GbACC_ACCrntUnctrolFlt_flg/1  "GbACC_ACCrntUnctrolFlt_flg"
  BMSDebounceStartZero/1 -> ACC_GbACC_ACCrntUnctrolFlt_flg/1
  Constant2/1 -> BMSDebounceStartZero/4
  Constant3/1 -> BMSDebounceStartZero/3
  Constant13/1 -> BMSDebounceStartZero/5
  Constant9/1 -> BMSDebounceStartZero/2

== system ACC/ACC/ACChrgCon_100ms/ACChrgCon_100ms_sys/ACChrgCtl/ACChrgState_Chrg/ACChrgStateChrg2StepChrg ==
  GcACC_ACChrgCrntRqst_A : Inport
  GcCDP_MaxCellVolt_mV : Inport  Port=2
  GeBTM_HeatReq_enum : Inport  Port=3
  GcUDS_FullChrgCutoffVolt_mV : Inport  Port=4
  Add : Sum  Inputs=+-
  BMSDebounceStartZero : AIWAYS_Powertrain_BMS_lib/Debounce & Delay/BMSDebounceStartZero
  Constant1 : Constant  Value=CcACC_ChrgSt2StepChrgTime_ms
  Constant11 : Constant  Value=ACC_RUNTIME_MS
  Constant2 : Constant  Value=CcACC_ChrgSt2StepChrgDeviVol_mV
  Constant3 : Constant  Value=Enum_BTMHeatReq.Enum_BTMHeatReq_Default
  Constant5 : Constant  Value=CcACC_ChrgStFullChrgCrnt_A
  Constant6 : Constant  Value=CcACC_ChrgSt2StepChrgTime_ms
  Constant9 : Constant  Value=ACC_RUNTIME_MS
  Data Type Conversion4 : DataTypeConversion
  Display{,1..4} (5 alike) : Display
  Logical Operator : Logic  Inputs=3  AllPortsSameDT=off  OutDataTypeStr=boolean
  Relational Operator : RelationalOperator  OutDataTypeStr=boolean
  Relational Operator1 : RelationalOperator  Operator===  OutDataTypeStr=boolean
  Relational Operator3 : RelationalOperator  Operator=>  OutDataTypeStr=boolean
  Scope : Scope
  LbACC_ChrgSt2StepChrg_flg : Outport
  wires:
  GcCDP_MaxCellVolt_mV/1 -> Display2/1, Relational Operator/1
  Constant5/1 -> Display1/1, Relational Operator3/2
  Relational Operator3/1 -> Logical Operator/1
  GcUDS_FullChrgCutoffVolt_mV/1 -> Add/1
  Logical Operator/1 -> BMSDebounceStartZero/1
  Relational Operator/1 -> Logical Operator/2
  GcACC_ACChrgCrntRqst_A/1 -> Display/1, Relational Operator3/1
  Relational Operator1/1 -> Display3/1, Logical Operator/3
  Constant3/1 -> Relational Operator1/2
  GeBTM_HeatReq_enum/1 -> Data Type Conversion4/1
  Data Type Conversion4/1 -> Relational Operator1/1
  BMSDebounceStartZero/1 -> Scope/1, Display4/1, LbACC_ChrgSt2StepChrg_flg/1  "LbACC_ChrgSt2StepChrg_flg"
  Constant6/1 -> BMSDebounceStartZero/4
  Constant1/1 -> BMSDebounceStartZero/2
  Constant9/1 -> BMSDebounceStartZero/5
  Constant11/1 -> BMSDebounceStartZero/3
  Add/1 -> Relational Operator/2
  Constant2/1 -> Add/2
